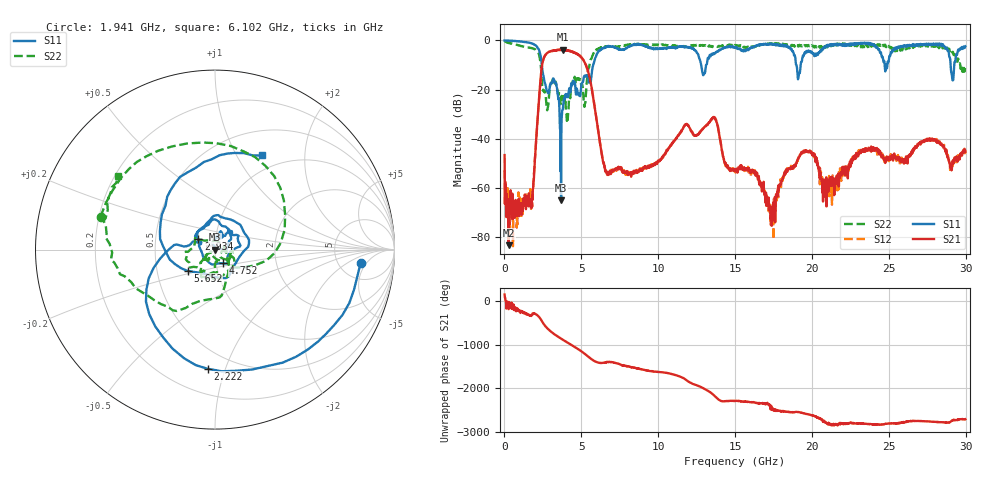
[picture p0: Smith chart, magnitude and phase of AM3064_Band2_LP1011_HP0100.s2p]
# Hz S DB R 50.0
!freq dBS11 angS11 dBS21 angS21 dBS12 angS12 dBS22 angS22
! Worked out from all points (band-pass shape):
!   1600 points, 10 MHz to 29.98 GHz, reference 50 ohm
!   highest |S21| = -3.76 dB at 3.777 GHz (marker M1); lowest = -83.2 dB at 272.4 MHz (marker M2)
!   |S21| within 3 dB of the highest: 2.587 GHz to 4.977 GHz (2.39 GHz wide, 63.2 % of centre)
!   lowest |S11| = -65.0 dB at 3.684 GHz (marker M3), VSWR 1.00, Z = 50 - j0.0414 ohm
!   |S11| at or under -10 dB: 2.426 GHz to 5.772 GHz (3.346 GHz wide, 81.6 % of centre); 12.8 GHz to 13.11 GHz (315.7 MHz wide, 2.44 % of centre); 18.98 GHz to 19.27 GHz (282.2 MHz wide, 1.48 % of centre)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
!   |S22| runs from -32.7 to -0.2 dB; largest |S21 - S12| = 0.019
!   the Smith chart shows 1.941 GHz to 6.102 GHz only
!   S11 on the Smith chart (normalised r, x): 1.941 GHz: 8.17, -3.61; 2.222 GHz: 0.37, -0.87; 2.934 GHz: 0.83, +0.10; 4.752 GHz: 1.08, -0.17; 5.652 GHz: 0.72, -0.18; 6.102 GHz: 0.80, +1.29
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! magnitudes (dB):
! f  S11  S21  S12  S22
! 10 MHz  0.0  -46.5  -52.7  -0.2
! 272.4 MHz  -0.1  -83.2  -62.3  -1.1
! 1.659 GHz  -1.0  -66.1  -65.5  -3.0
! 1.941 GHz  -1.8  -52.2  -52.8  -3.6
! 2.222 GHz  -3.5  -26.2  -26.0  -5.3
! 2.934 GHz  -19.3  -4.6  -4.6  -20.1
! 3.684 GHz  -65.0  -3.9  -3.7  -23.1
! 3.777 GHz  -28.2  -3.8  -3.9  -24.7
! 4.752 GHz  -21.1  -5.6  -5.6  -15.9
! 5.015 GHz  -17.6  -7.0  -7.0  -18.5
! 5.652 GHz  -14.3  -18.5  -18.5  -7.4
! 6.102 GHz  -4.6  -36.9  -36.8  -3.4
! 6.683 GHz  -2.6  -54.1  -54.6  -2.5
! 10 GHz  -3.4  -48.8  -49.2  -1.9
! 13.6 GHz  -5.4  -31.6  -31.5  -2.5
! 15 GHz  -2.7  -53.1  -52.5  -1.9
! 16.35 GHz  -2.4  -53.7  -53.7  -2.6
! 17.35 GHz  -1.4  -69.6  -72.1  -1.2
! 19.99 GHz  -4.7  -46.1  -45.9  -2.0
! 20.87 GHz  -2.3  -63.5  -59.3  -2.9
! 25 GHz  -8.3  -48.5  -47.5  -2.2
! 29.98 GHz  -2.4  -45.2  -45.6  -10.3
